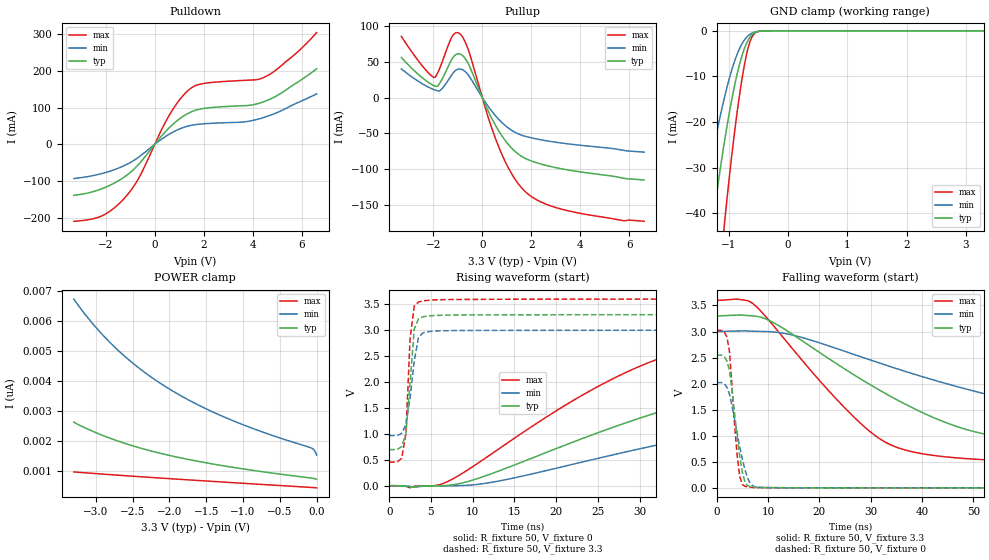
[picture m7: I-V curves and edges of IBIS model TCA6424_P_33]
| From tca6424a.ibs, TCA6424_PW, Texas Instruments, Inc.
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[Model]   TCA6424_P_33
Model_type  I/O
Vinl=0.9
Vinh=2.52
Enable   Active-Low
Vref =   0
Rref =   500
Cref =   50p
Vmeas =   1.65
| variable   typ   min   max
C_comp   3.67pF   2.94pF   4.06pF
| C_pullup   6.91pF   2.70pF   10.67pF
| C_pulldown   4.38pF   3.36pF   6.01pF
| C_tri-state   3.67pF   2.94pF   4.06pF
[Temperature Range]   40   100   -40
| Ambient temperature   25   85   -40
[Voltage range]   3.3   3   3.6
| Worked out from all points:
|   slope of the pulldown table from 0 to 0.495 V, typ, clamps not added: 12.8 ohm
|   slope of the pullup table from 0 to 0.495 V, typ, clamps not added: 13.7 ohm
|   GND clamp passes 1 mA (typ) near -0.61 V on its own axis
|   rising waveform, R_fixture 50, V_fixture 0: 20-80 % time 30.7ns typ, 44.3ns min, 19.6ns max; typ from 0 V to 2.55 V
|   falling waveform, R_fixture 50, V_fixture 3.3: 20-80 % time 28.3ns typ, 48.6ns min, 17.6ns max; typ from 3.3 V to 0.697 V
|   rising waveform, R_fixture 50, V_fixture 3.3: 20-80 % time 771ps typ, 1.01ns min, 585ps max; typ from 0.697 V to 3.3 V
|   falling waveform, R_fixture 50, V_fixture 0: 20-80 % time 1.86ns typ, 2.47ns min, 1.36ns max; typ from 2.55 V to 0 V
[GND Clamp]
| TCA6424_P_33
|   Voltage   I(typ)   I(min)   I(max)
-3.3V     -320.1mA   -236mA     -448.8mA
-1.475V   -64.16mA   -42.41mA   -102.7mA
-1.285V   -43.97mA   -28.12mA   -72.67mA
-1.255V   -41mA      -26.05mA   -68.18mA
-1.08V    -25.17mA   -15.22mA   -43.69mA
-1.055V   -23.14mA   -13.86mA   -40.46mA
-930mV    -14mA      -7.921mA   -25.56mA
-795mV    -6.402mA   -3.374mA   -12.33mA
-695mV    -2.699mA   -1.399mA   -5.04mA
-600mV    -817.7uA   -469.8uA   -1.244mA
-405mV    -18.71uA   -16.33uA   -14.76uA
3.3V      709.5pA    1.936nA    -452.1pA
[POWER Clamp]
| TCA6424_P_33
|   Voltage   I(typ)   I(min)   I(max)
-3.3V     2.622nA    6.737nA    956.4pA
-3.18V    2.469nA    6.332nA    933.6pA
-3.04V    2.312nA    5.907nA    907.7pA
-2.75V    2.032nA    5.146nA    856.1pA
-2.435V   1.783nA    4.47nA     802.5pA
-2.09V    1.56nA     3.867nA    746.1pA
-1.685V   1.346nA    3.291nA    681.9pA
-1.225V   1.145nA    2.76nA     610.8pA
-720mV    958.2pA    2.279nA    534.2pA
-70mV     749.4pA    1.754nA    436.6pA
-30mV     732.7pA    1.676nA    429.7pA
-48.03fV  709.5pA    1.52nA     423.6pA
[Pulldown]
| TCA6424_P_33
|   Voltage   I(typ)   I(min)   I(max)
-3.3V     -138.9mA   -93.2mA    -209.6mA
-2.145V   -120.7mA   -79.32mA   -194.6mA
-1.205V   -87.25mA   -56.7mA    -144.4mA
-625mV    -52.16mA   -33.29mA   -88.82mA
635mV     48.12mA    29.38mA    84.09mA
1.045V    71.26mA    42.81mA    124.1mA
1.44V     87.04mA    51.09mA    151.2mA
2.03V     98.12mA    56.17mA    166.2mA
3.635V    105.3mA    60.96mA    174.2mA
4.46V     116.4mA    73.47mA    182.6mA
5.665V    162.5mA    108.5mA    242.4mA
6.6V      205.7mA    137.4mA    304.5mA
[Pullup]
| TCA6424_P_33
|   Voltage   I(typ)   I(min)   I(max)
-3.3V     55.99mA    39.93mA    85.31mA
-1.95V    16.25mA    10.75mA    28.04mA
-1.695V   22.09mA    10.36mA    44.17mA
-1.215V   54.77mA    33mA       85.82mA
-855mV    59.88mA    39.51mA    86.91mA
-550mV    45.78mA    30.48mA    64.67mA
240mV     -18.75mA   -12.28mA   -27.4mA
755mV     -51.07mA   -33.38mA   -75.76mA
1.325V    -74.85mA   -48.35mA   -113.4mA
1.915V    -87.39mA   -55.54mA   -136mA
3.535V    -101.3mA   -64.82mA   -158.4mA
6.6V      -115.1mA   -76.16mA   -172.7mA
[Ramp]
| TCA6424_P_33
| variable   typ   min   max
dV/dt_r   1.55/3.10E-08   1.23/4.45E-08   1.84/1.98E-08
dV/dt_f   1.57/2.84E-08   1.23/4.87E-08   1.90/1.77E-08
R_load = 50
[Rising Waveform]
| TCA6424_P_33
R_fixture =   50
C_fixture =   0
L_fixture =   0
V_fixture =   0
V_fixture_min = 0
V_fixture_max = 0
|   Time   V(typ)   V(min)   V(max)
0s        2.1nV      15.64nV    590pV
7ns       5.109mV    -2.06mV    79.96mV
12.5ns    245.4mV    71.48mV    639.3mV
23ns      901.4mV    451.3mV    1.734V
33.5ns    1.481V     832.5mV    2.516V
41.5ns    1.831V     1.083V     2.779V
55ns      2.217V     1.417V     2.923V
84.5ns    2.459V     1.817V     3.001V
132.5ns   2.532V     1.975V     3.022V
520ns     2.547V     2.019V     3.025V
[Falling Waveform]
| TCA6424_P_33
R_fixture =   50
C_fixture =   0
L_fixture =   0
V_fixture =   3.3
V_fixture_min = 3
V_fixture_max = 3.6
|   Time   V(typ)   V(min)   V(max)
0s        3.3V       3V         3.6V
7.5ns     3.296V     3.005V     3.499V
23ns      2.404V     2.685V     1.735V
32ns      1.858V     2.385V     926mV
38.5ns    1.518V     2.18V      683.6mV
50ns      1.083V     1.859V     552.1mV
63ns      880.4mV    1.566V     501.4mV
83.5ns    771.7mV    1.263V     472.4mV
131ns     710.7mV    1.039V     457.3mV
520ns     697.3mV    967.8mV    455mV
[Rising Waveform]
| TCA6424_P_33
R_fixture =   50
C_fixture =   0
L_fixture =   0
V_fixture =   3.3
V_fixture_min = 3
V_fixture_max = 3.6
|   Time   V(typ)   V(min)   V(max)
0s        697.3mV    967.8mV    455mV
1ns       702.4mV    968.2mV    463.7mV
1.5ns     757.3mV    1.01V      529mV
2ns       996mV      1.174V     1.001V
2.5ns     1.983V     1.691V     2.837V
3ns       3.022V     2.408V     3.463V
3.5ns     3.219V     2.857V     3.543V
4ns       3.258V     2.944V     3.564V
5.5ns     3.284V     2.983V     3.586V
520ns     3.3V       3V         3.6V
[Falling Waveform]
| TCA6424_P_33
R_fixture =   50
C_fixture =   0
L_fixture =   0
V_fixture =   0
V_fixture_min = 0
V_fixture_max = 0
|   Time   V(typ)   V(min)   V(max)
0s        2.547V     2.019V     3.025V
1.5ns     2.514V     1.994V     2.986V
2ns       2.434V     1.929V     2.894V
2.5ns     2.252V     1.795V     2.606V
3.5ns     1.408V     1.304V     1.188V
4ns       966.4mV    1.038V     602.8mV
4.5ns     588.6mV    781mV      214mV
5.5ns     114.9mV    349.7mV    30.12mV
7ns       15.27mV    36.31mV    8.748mV
520ns     71.09nV    281.5nV    38.79nV
